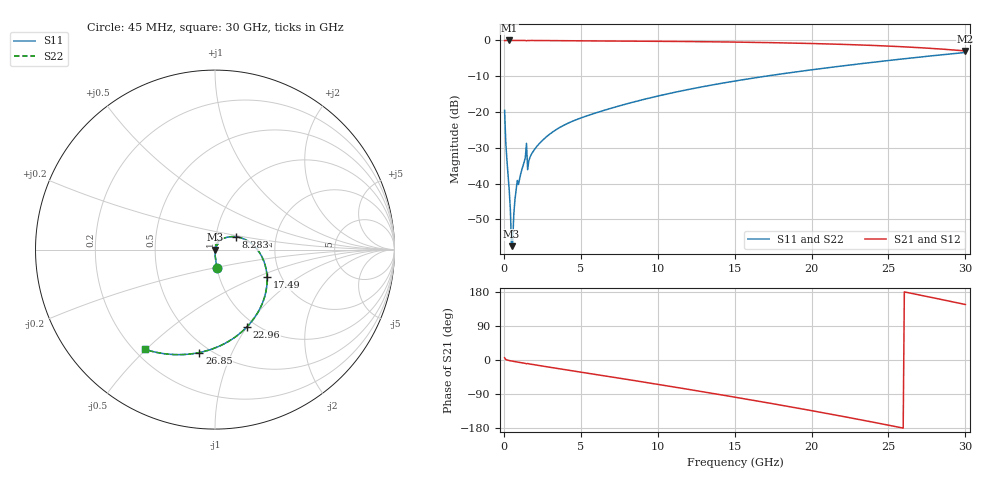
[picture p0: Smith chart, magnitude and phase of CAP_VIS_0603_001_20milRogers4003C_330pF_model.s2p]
! S-parameter model data by Modelithics Inc.  support@modelithics.com  813-866-6335  Tampa FL USA
! S-Parameter data specifications:
! Substrate: 20-mil Rogers 4003C, substrate thickness, H=0.508mm, Dielectric constant, Er=3.75
! PCB Mounting Pad Footprint: Pad width, PadW=0.90mm , Pad length, PadL=1.00mm , Pad gap, PadG (edge-to-edge)=1.00mm , Reference planes=3.0mm apart
! Created Wed Nov 18 13:34:03 2015
# hz S ma R 50
! 2 Port Network Data from SP1.SP block
! freq  magS11  angS11  magS21  angS21  magS12  angS12  magS22  angS22
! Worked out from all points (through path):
!   401 points, 45 MHz to 30 GHz, reference 50 ohm
!   highest |S21| = 0.00 dB at 344.6 MHz (marker M1); lowest = -2.9 dB at 30 GHz (marker M2)
!   group delay of S21, straight-line fit = 19.6 ps
!   lowest |S11| = -57.5 dB at 494.3 MHz (marker M3), VSWR 1.00, Z = 50 - j0.126 ohm
!   |S11| at or under -10 dB: start of sweep to 17.01 GHz
!   |S22| runs from -57.5 to -3.4 dB; largest |S21 - S12| = 0
!   S11 on the Smith chart (normalised r, x): 45 MHz: 1.00, -0.21; 8.283 GHz: 1.24, +0.18; 17.49 GHz: 1.69, -0.58; 22.96 GHz: 0.91, -1.00; 26.85 GHz: 0.44, -0.76; 30 GHz: 0.24, -0.50
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4.5e7  0.1055 -84.1  0.9942 5.8  0.9942 5.8  0.1055 -84.1
1.94775e8  0.02138 -88.9  0.9994 0.2  0.9994 0.2  0.02138 -88.9
3.4455e8  0.008087 -88.4  0.9995 -1.4  0.9995 -1.4  0.008087 -88.4
4.194375e8  0.004311 -85.9  0.9995 -2.1  0.9995 -2.1  0.004311 -85.9
4.94325e8  0.001334 -70.7  0.9995 -2.6  0.9995 -2.6  0.001334 -70.7
6.441e8  0.003778 77.5  0.9994 -3.7  0.9994 -3.7  0.003778 77.5
7.93875e8  0.008239 80.0  0.9992 -4.8  0.9992 -4.8  0.008239 80.0
8.687625e8  0.01105 77.8  0.9985 -5.4  0.9985 -5.4  0.01105 77.8
1.318088e9  0.02003 78.7  0.9986 -8.4  0.9986 -8.4  0.02003 78.7
1.692525e9  0.02322 76.6  0.9985 -10.6  0.9985 -10.6  0.02322 76.6
2.14185e9  0.03307 73.9  0.9978 -13.6  0.9978 -13.6  0.03307 73.9
3.115388e9  0.05158 66.2  0.995 -20.0  0.995 -20.0  0.05158 66.2
5.062462e9  0.08343 50.8  0.9863 -32.4  0.9863 -32.4  0.08343 50.8
8.282625e9  0.1353 31.9  0.9782 -53.0  0.9782 -53.0  0.1353 31.9
1.007992e10  0.1685 21.2  0.9729 -64.8  0.9729 -64.8  0.1685 21.2
1.50225e10  0.271 -10.7  0.9488 -98.1  0.9488 -98.1  0.271 -10.7
1.749379e10  0.3276 -27.7  0.9304 -115.5  0.9304 -115.5  0.3276 -27.7
2.003996e10  0.3896 -45.9  0.9056 -133.9  0.9056 -133.9  0.3896 -45.9
2.296058e10  0.4664 -67.7  0.868 -156.0  0.868 -156.0  0.4664 -67.7
2.505742e10  0.526 -84.1  0.8329 -172.5  0.8329 -172.5  0.526 -84.1
2.685472e10  0.5799 -98.6  0.7961 172.9  0.7961 172.9  0.5799 -98.6
3e10  0.6788 -125.0  0.7138 146.4  0.7138 146.4  0.6788 -125.0
